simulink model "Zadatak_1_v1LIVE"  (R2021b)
settings: Solver=VariableStepAuto  StartTime=0.0  StopTime=0.1  RelTol=1e-3
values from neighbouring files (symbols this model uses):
  f = 50    [Script_Zad_1.m]    (also in Script_Zad_1_Nominal.m)
  Rl = 3    [Script_Zad_1.m]    (also in Script_Zad_1_Nominal.m)
  Uab = 380    [Script_Zad_1.m]    (also in Script_Zad_1_Nominal.m)
libraries: spsThreePhaseVIMeasurementLib x3, spsThreePhaseSeriesRLCLoadLib x2, spsPower3phInstantaneousLib x2, spsRMSLib x1, spsThreePhaseSeriesRLCBranchLib x1, spsSequenceAnalyzerLib x1, spsThreePhaseSourceLib x1, spspowerguiLib x1

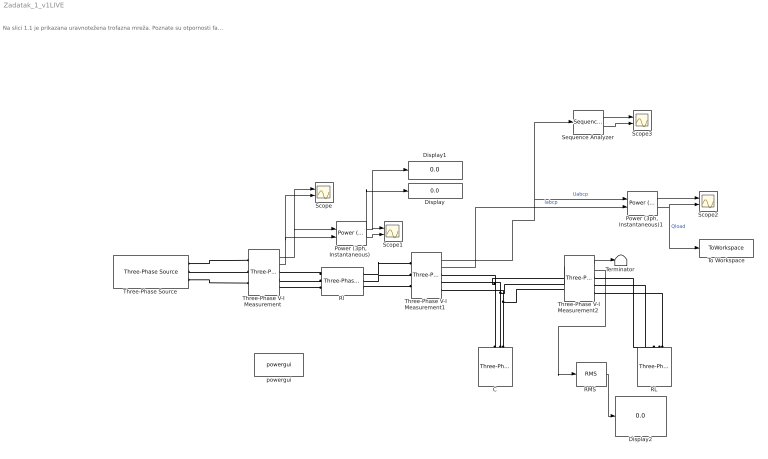
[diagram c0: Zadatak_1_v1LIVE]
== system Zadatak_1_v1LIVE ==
  note: Na slici 1.1 je prikazana uravnotežena trofazna mreža. Poznate su otpornosti faznih provodnika, 𝑅𝑙 , kao i parametri prijemnika (elektromotora) vezanog u zvezdu: 𝑅 i 𝐿 . Mreža se napaja linijskim naponima koji obrazuju simetričan direktan sistem prvog reda efektivne vrednosti 𝑈 i frekvencije 𝑓 = 𝜔 2𝜋 . Odrediti (a) kapacitivnosti kondenzatora 𝐶, koje treba vezati u trougao na krajevima prijemnika, kako bi faktor snage mreže bio maksimalan, (b) aktivnu snagu mreže i prijemnika pri ispunjenom uslovu pod (a) i (c) fazorski dijagram napona mreže pri ispunjenom uslovu pod (a). Brojne vrednosti: 𝑈 = 380 V, 𝑓 = 50 Hz, 𝑅𝑙 = 3 Ω, 𝑅 = 20 Ω, 𝐿 = 50 mH.
  C : spsThreePhaseSeriesRLCLoadLib/Three-Phase Series RLC Load  LConnTagsString=A|B|C  Configuration=Delta  NominalVoltage=Unom  Vabc=[1e3 1e3 1e3]  Vabcp=[1e3 1e3 1e3]  NominalFrequency=f  UnbalancedPower=off  ActivePower=0  InductivePower=0  CapacitivePower=QC  Pabc=[10e3 9e3 11e3]  QLabc=[100 90 110]  QCabc=[100 90 110]  Pabcp=[10e3 9e3 11e3]  QLabcp=[100 90 110]  QCabcp=[100 90 110]  Measurements=None  LoadType=constant Z
  Display : Display
  Display1 : Display
  Display2 : Display
  "Power (3ph, Instantaneous) " : spsPower3phInstantaneousLib/Power (3ph, Instantaneous)
  "Power (3ph, Instantaneous)1 " : spsPower3phInstantaneousLib/Power (3ph, Instantaneous)
  RL : spsThreePhaseSeriesRLCLoadLib/Three-Phase Series RLC Load  LConnTagsString=A|B|C  Configuration=Y (grounded)  NominalVoltage=Unom  Vabc=[1e3 1e3 1e3]  Vabcp=[1e3 1e3 1e3]  NominalFrequency=f  UnbalancedPower=off  ActivePower=PR  InductivePower=QL  CapacitivePower=0  Pabc=[10e3 9e3 11e3]  QLabc=[100 90 110]  QCabc=[100 90 110]  Pabcp=[10e3 9e3 11e3]  QLabcp=[100 90 110]  QCabcp=[100 90 110]  Measurements=None  LoadType=constant Z
  "RMS " : spsRMSLib/RMS  TrueRMS=on  Freq=f  RMSInit=0  Ts=0
  Rl : spsThreePhaseSeriesRLCBranchLib/Three-Phase Series RLC Branch  LConnTagsString=A|B|C  RConnTagsString=A|B|C  BranchType=R  Resistance=Rl  Inductance=0  Capacitance=0  Measurements=None
  Scope{,1..3} (4 alike) : Scope  NumInputPorts=2
  "Sequence Analyzer " : spsSequenceAnalyzerLib/Sequence Analyzer  Freq=f  n=1  seq=Positive Negative Zero  InInit=[1, 0]  Ts=0
  "Terminator " : Terminator
  "Three-Phase V-I Measurement " : spsThreePhaseVIMeasurementLib/Three-Phase V-I Measurement  VoltageMeasurement=phase-to-ground  SetLabelV=off  LabelV=Vabc  Vpu=off  VpuLL=off  CurrentMeasurement=yes  SetLabelI=off  LabelI=Iabc  Ipu=off  Pbase=100e6  Vbase=500e3  OutputType=Complex  PhasorSimulation=off  PSBequivalent=0
  "Three-Phase V-I Measurement1 " : spsThreePhaseVIMeasurementLib/Three-Phase V-I Measurement  VoltageMeasurement=phase-to-ground  SetLabelV=off  LabelV=Vabc  Vpu=off  VpuLL=off  CurrentMeasurement=yes  SetLabelI=off  LabelI=Iabc  Ipu=off  Pbase=100e6  Vbase=500e3  OutputType=Complex  PhasorSimulation=off  PSBequivalent=0
  "Three-Phase V-I Measurement2 " : spsThreePhaseVIMeasurementLib/Three-Phase V-I Measurement  VoltageMeasurement=phase-to-ground  SetLabelV=off  LabelV=Vabc  Vpu=off  VpuLL=off  CurrentMeasurement=yes  SetLabelI=off  LabelI=Iabc  Ipu=off  Pbase=100e6  Vbase=500e3  OutputType=Complex  PhasorSimulation=off  PSBequivalent=0
  "Three-Phase Source " : spsThreePhaseSourceLib/Three-Phase Source  InternalConnection=Yg  VoltagePhases=off  Voltage=Uab  PhaseAngle=0  Voltage_phases=[25e3 25e3 25e3]/sqrt(3)  PhaseAngles_phases=[0 -120 +120]  Frequency=f  NonIdealSource=off  SpecifyImpedance=off  Resistance=0.8929  Inductance=16.58e-3  ShortCircuitLevel=100e6  BaseVoltage=25e3  XRratio=7  BusType=swing  Pref=10e3  Qref=0  Prefabc=[10e3, 10e3, 10e3]  Qrefabc=[0, 0, 0]  Qmin=-inf  Qmax=inf
  To Workspace : ToWorkspace  VariableName=Qload  SaveFormat=Timeseries  SampleTime=-1
  powergui : spspowerguiLib/powergui  Priority=1  SimulationMode=Continuous  SampleTime=50e-6  frequency=60  Iterations=50  frequencyindice=50  Pbase=100e6  ErrMax=1e-4  UnitsV=kV  UnitsW=MW  buscounter=0  FunctionMessages=off  echomessages=off  EnableUseOfTLC=off  CurrentSourceSwitches=off  DisableSnubberDevices=off  DisableRonSwitches=off  DisableVfSwitches=off  DisplayEquations=off  AutomaticDiscreteSolvers=off  SolverType=Tustin/Backward Euler (TBE)  Interpol=off  ExternalGateDelay=off  methode=off  Ts=100  x0status=blocks  SPID=on  SwTol=0  HookPort=off  NonlinearTolerance=1e-4  nMaxIteration=100  ContinueOnMaxIteration=off  RestoreLinks=warning  ResistiveCurrentMeasurement=off  Frange=[0:2:500]  Ylog=off  Xlog=on  ShowGrid=off  save=off  variable=ZData  structure=0  ZoomFFT=off  StartTime=0.0  cycles=1  DisplayStyle=1  fundamental=60  FreqAxis=off  MaxFrequency=1000  frequencyindicesteady=1  RmsSteady=1  display=off
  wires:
  "Three-Phase V-I Measurement "/1 -> "Power (3ph, Instantaneous) "/1, Scope/1
  "Three-Phase V-I Measurement "/2 -> "Power (3ph, Instantaneous) "/2, Scope/2
  "Power (3ph, Instantaneous) "/1 -> Display1/1, Scope1/1
  "Power (3ph, Instantaneous) "/2 -> Display/1, Scope1/2
  "Power (3ph, Instantaneous)1 "/1 -> Scope2/1
  "Power (3ph, Instantaneous)1 "/2 -> To Workspace/1, Scope2/2  "Qload"
  "Three-Phase V-I Measurement1 "/1 -> "Sequence Analyzer "/1, "Power (3ph, Instantaneous)1 "/1  "Uabcp"
  "Three-Phase V-I Measurement1 "/2 -> "Power (3ph, Instantaneous)1 "/2  "Iabcp"
  "Sequence Analyzer "/1 -> Scope3/1
  "Sequence Analyzer "/2 -> Scope3/2
  "Three-Phase V-I Measurement2 "/2 -> "RMS "/1
  "RMS "/1 -> Display2/1
  "Three-Phase V-I Measurement2 "/1 -> "Terminator "/1
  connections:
  C/LConn1 -- "Three-Phase V-I Measurement2 "/LConn1 -- "Three-Phase V-I Measurement1 "/RConn1
  C/LConn2 -- "Three-Phase V-I Measurement2 "/LConn2 -- "Three-Phase V-I Measurement1 "/RConn2
  C/LConn3 -- "Three-Phase V-I Measurement2 "/LConn3 -- "Three-Phase V-I Measurement1 "/RConn3
  Rl/LConn1 -- "Three-Phase V-I Measurement "/RConn1
  "Three-Phase V-I Measurement "/RConn2 -- Rl/LConn2
  Rl/LConn3 -- "Three-Phase V-I Measurement "/RConn3
  "Three-Phase Source "/RConn3 -- "Three-Phase V-I Measurement "/LConn3
  "Three-Phase Source "/RConn2 -- "Three-Phase V-I Measurement "/LConn2
  "Three-Phase Source "/RConn1 -- "Three-Phase V-I Measurement "/LConn1
  Rl/RConn1 -- "Three-Phase V-I Measurement1 "/LConn1
  Rl/RConn2 -- "Three-Phase V-I Measurement1 "/LConn2
  Rl/RConn3 -- "Three-Phase V-I Measurement1 "/LConn3
  "Three-Phase V-I Measurement2 "/RConn1 -- RL/LConn1
  "Three-Phase V-I Measurement2 "/RConn2 -- RL/LConn2
  RL/LConn3 -- "Three-Phase V-I Measurement2 "/RConn3
